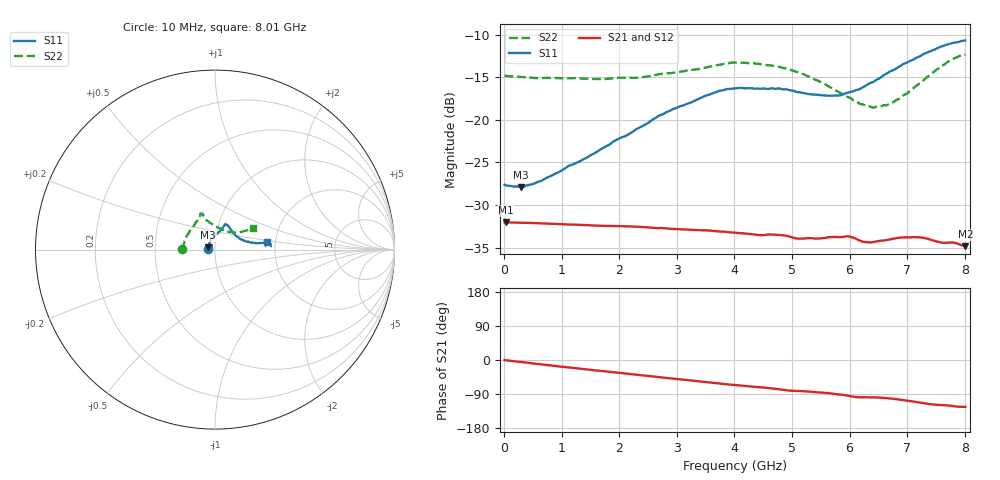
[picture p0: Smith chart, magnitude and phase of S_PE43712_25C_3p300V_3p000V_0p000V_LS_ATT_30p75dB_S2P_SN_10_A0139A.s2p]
! DEVICE ID: PE43712
! File Path: z:\PE43713\PE43713_CHAR_NOM_04292014\AMB\3p300\LS_ATT_30p75dB\PE43713_AMB_3p300V_3p000V_0p000V_LS_ATT_30p75dB_S2P_SN_10_A0139A.s2p
! Serial: 10
! Lot: A0139A
! Temp: 25C
! VDD: 3.300
! VSS: 0.000
! Control_Hi: 3.000
! Control_Lo: 0.000
! Attenuation Step: 30.75dB
! Port 1: RF1
! Port 2: RF2
! ThroughPath:1-2
! IDD: 0.0001457545
! ISS: -1.569e-007
#  Hz  S  RI  R  50
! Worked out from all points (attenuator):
!   801 points, 10 MHz to 8.01 GHz, reference 50 ohm
!   highest |S21| = -32.02 dB at 30 MHz (marker M1); lowest = -34.8 dB at 8.01 GHz (marker M2)
!   lowest |S11| = -27.9 dB at 290 MHz (marker M3), VSWR 1.08, Z = 46.3 + j1.23 ohm
!   |S11| at or under -10 dB: start of sweep to end of sweep
!   |S22| runs from -18.6 to -12.3 dB; largest |S21 - S12| = 0.00011
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1e7  -0.0416 0.000894  0.025 -0.000114  0.0251 -0.000102  -0.1814 0.0012
3e7  -0.0412 0.00221  0.025 -0.00025  0.0251 -0.000258  -0.1809 0.0029
2.9e8  -0.0381 0.0133  0.0248 -0.00233  0.0248 -0.00233  -0.1773 0.0185
6.5e8  -0.0338 0.0281  0.0242 -0.00499  0.0242 -0.005  -0.1711 0.0393
1.35e9  -0.021 0.054  0.0222 -0.00962  0.0222 -0.00963  -0.1568 0.0766
2.31e9  0.0103 0.0881  0.0183 -0.0149  0.0183 -0.0149  -0.1226 0.1267
2.68e9  0.025 0.1023  0.0164 -0.0164  0.0164 -0.0164  -0.1069 0.1511
3.5e9  0.0484 0.1298  0.0119 -0.0191  0.0119 -0.0191  -0.0838 0.1842
3.74e9  0.0533 0.138  0.0104 -0.0196  0.0104 -0.0196  -0.0815 0.1941
4.01e9  0.0582 0.1415  0.00881 -0.0199  0.00881 -0.0199  -0.0806 0.2013
4.76e9  0.0721 0.1345  0.00473 -0.0206  0.00475 -0.0206  -0.0665 0.1941
5.1e9  0.0825 0.1195  0.00289 -0.0199  0.0029 -0.0199  -0.0585 0.181
5.35e9  0.0911 0.1073  0.00202 -0.0201  0.00204 -0.0201  -0.0513 0.1683
5.82e9  0.1143 0.0792  -0.000342 -0.0205  -0.000336 -0.0206  -0.0196 0.1432
5.99e9  0.1269 0.0704  -0.00174 -0.0207  -0.00171 -0.0206  -0.00425 0.1351
6.2e9  0.1414 0.0584  -0.00288 -0.0192  -0.0028 -0.0192  0.0177 0.1221
6.41e9  0.1583 0.0514  -0.00275 -0.019  -0.00268 -0.019  0.0413 0.1104
6.68e9  0.1852 0.0435  -0.00381 -0.0195  -0.00379 -0.0195  0.0737 0.0993
6.88e9  0.2029 0.0386  -0.00523 -0.0197  -0.00516 -0.0197  0.0944 0.0952
7.22e9  0.2329 0.0354  -0.00777 -0.0189  -0.00773 -0.0188  0.1323 0.0966
7.7e9  0.274 0.0391  -0.00949 -0.0165  -0.00944 -0.0165  0.1883 0.1101
8.01e9  0.2886 0.0432  -0.0101 -0.0151  -0.00998 -0.0151  0.2112 0.1177
